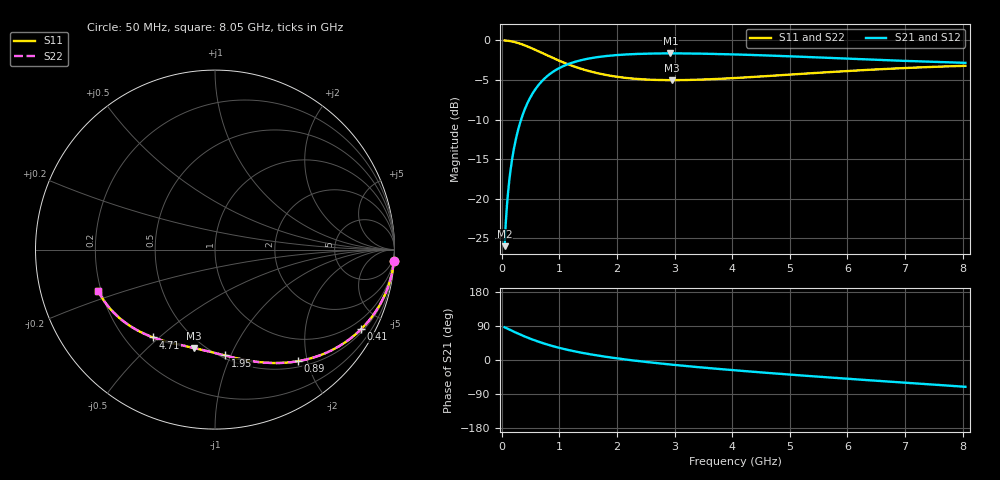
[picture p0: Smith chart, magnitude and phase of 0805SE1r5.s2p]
! AVX Thin Film Operation		Date: August 2001
! Description: Accu-P® Series, Thin Film, SMD, RF Capacitor
! Part Number: 08051J1R5ABT
! 50 MHz  -  8.05 GHz
! Serial Measurements
# mhz S db R 50
!	S11		S21		S12		S22
!	dB	Phase	dB	Phase	dB	Phase	dB	Phase
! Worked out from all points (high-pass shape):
!   401 points, 50 MHz to 8.05 GHz, reference 50 ohm
!   highest |S21| = -1.65 dB at 2.93 GHz (marker M1); lowest = -26.0 dB at 50 MHz (marker M2)
!   |S21| within 3 dB of the highest: 769.4 MHz to end of sweep
!   lowest |S11| = -5.0 dB at 2.95 GHz (marker M3), VSWR 3.55, Z = 22.1 - j35.4 ohm
!   |S11| at or under -10 dB: nowhere
!   |S22| runs from -5.0 to 0.0 dB; largest |S21 - S12| = 0
!   S11 on the Smith chart (normalised r, x): 50 MHz: 1, -31; 410 MHz: 0.61, -3.84; 890 MHz: 0.59, -1.83; 1.95 GHz: 0.52, -0.95; 4.71 GHz: 0.31, -0.48; 8.05 GHz: 0.19, -0.17
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50  -0.01 -3.7  -26.00 86.3  -26.00 86.3  -0.01 -3.7
70  -0.02 -5.1  -23.09 84.9  -23.09 84.9  -0.02 -5.1
130  -0.07 -9.5  -17.77 80.5  -17.77 80.5  -0.07 -9.5
190  -0.15 -13.8  -14.58 76.2  -14.58 76.2  -0.15 -13.8
290  -0.35 -20.7  -11.15 69.3  -11.15 69.3  -0.35 -20.7
410  -0.66 -28.5  -8.53 61.4  -8.53 61.4  -0.66 -28.6
510  -0.96 -34.6  -7.03 55.4  -7.03 55.4  -0.96 -34.6
630  -1.35 -41.2  -5.72 48.7  -5.72 48.7  -1.35 -41.3
890  -2.23 -53.5  -3.97 36.5  -3.97 36.5  -2.23 -53.5
1130  -2.96 -62.7  -3.06 27.3  -3.06 27.3  -2.96 -62.7
1390  -3.62 -70.9  -2.48 19.1  -2.48 19.1  -3.62 -70.9
1650  -4.12 -77.7  -2.13 12.2  -2.13 12.2  -4.12 -77.8
1950  -4.54 -84.5  -1.88 5.4  -1.88 5.4  -4.54 -84.6
2310  -4.85 -91.6  -1.73 -1.7  -1.73 -1.7  -4.85 -91.6
2730  -5.01 -98.7  -1.65 -8.8  -1.65 -8.8  -5.01 -98.8
2930  -5.03 -101.8  -1.65 -11.9  -1.65 -11.9  -5.03 -101.9
2950  -5.03 -102.1  -1.65 -12.2  -1.65 -12.2  -5.03 -102.2
4050  -4.76 -117.1  -1.78 -27.2  -1.78 -27.2  -4.76 -117.2
4710  -4.46 -125.1  -1.93 -35.2  -1.93 -35.2  -4.46 -125.1
5390  -4.14 -132.7  -2.12 -42.9  -2.12 -42.9  -4.14 -132.8
6730  -3.59 -147.0  -2.52 -57.1  -2.52 -57.1  -3.59 -147.0
8050  -3.21 -160.5  -2.84 -70.7  -2.84 -70.7  -3.21 -160.6
